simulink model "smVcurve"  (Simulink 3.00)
settings: Solver=ode45  StartTime=0.0  StopTime=0  MaxStep=3  RelTol=1e-3
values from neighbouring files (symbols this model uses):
  Ef = parEf(m)    [Ccurverun.m]
  Ra = .95    (= 0.95)    [altwdgs.m]    (also in Ccurverun.m = 0.018)
  Tl = Tl2    [calc0.m]
  Vs = abs(Vas)    [calc0.m]    (also in Ccurverun.m = 1; IMabc2.m = 1; IMabcrun0.m = Vll*sqrt(2/3); IMabcrun1.m = Vll*sqrt(2/3))
  Xd = 1.15    [Ccurverun.m]
  Xq = 0.75    [Ccurverun.m]
libraries: simulink3 x3

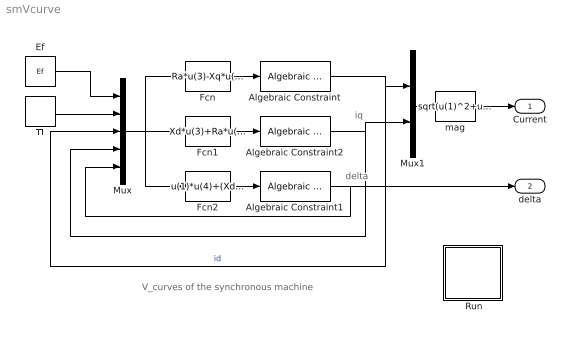
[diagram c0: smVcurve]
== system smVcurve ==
  note: iq
  note: delta
  note: V_curves of the synchronous machine
  " Run" : Subsystem
  Algebraic Constraint : simulink3/Math/Algebraic Constraint  z0=1
  Algebraic Constraint1 : simulink3/Math/Algebraic Constraint  z0=.1
  Algebraic Constraint2 : simulink3/Math/Algebraic Constraint  z0=1
  Ef : Constant  Value=Ef
  Fcn : Fcn  Expr=Ra*u(3)-Xq*u(4)+Vs*sin(u(5))
  Fcn1 : Fcn  Expr=Xd*u(3)+Ra*u(4)-Vs*cos(u(5))+u(1)
  Fcn2 : Fcn  Expr=u(1)*u(4)+(Xd-Xq)*u(3)*u(4)-u(2)
  Mux : Mux  Inputs=5
  Mux1 : Mux  Inputs=2
  Tl : Constant  Value=Tl
  mag : Fcn  Expr=sqrt(u(1)^2+u(2)^2)
  Current : Outport  Port=1
  delta : Outport  Port=2
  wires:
  Mux/1 -> Fcn1/1, Fcn2/1, Fcn/1
  Ef/1 -> Mux/1
  Tl/1 -> Mux/2
  Fcn/1 -> Algebraic Constraint/1
  Fcn1/1 -> Algebraic Constraint2/1
  Fcn2/1 -> Algebraic Constraint1/1
  Algebraic Constraint/1 -> Mux/3, Mux1/1  "id"
  Algebraic Constraint2/1 -> Mux/4, Mux1/2
  Algebraic Constraint1/1 -> Mux/5, delta/1
  Mux1/1 -> mag/1
  mag/1 -> Current/1

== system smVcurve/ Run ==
  note: Double click the block to enter the machine parameters and run the simulation
  note: This demo illustrates the generation of the V_ and C_curves of a synchronous machine
